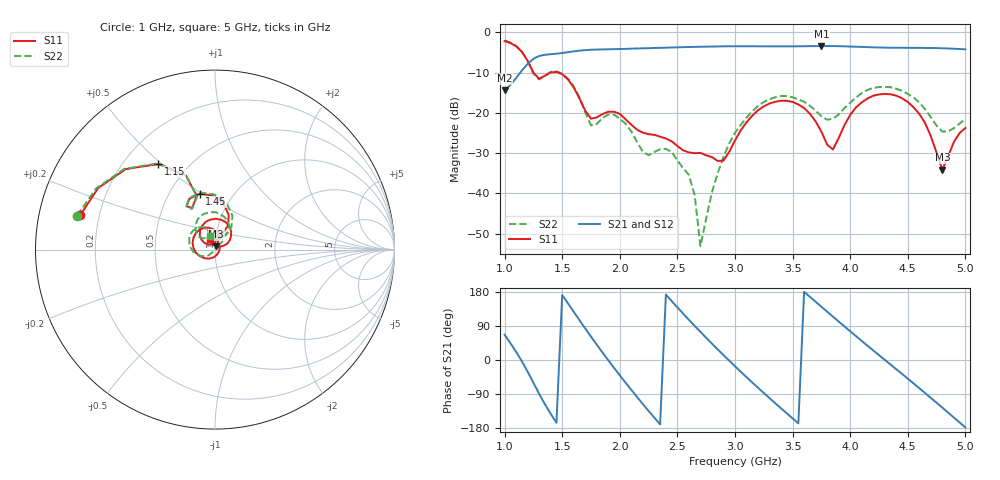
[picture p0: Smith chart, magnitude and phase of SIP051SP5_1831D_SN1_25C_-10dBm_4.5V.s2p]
# GHz  S  dB  R  50
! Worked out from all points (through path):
!   81 points, 1 GHz to 5 GHz, reference 50 ohm
!   highest |S21| = -3.41 dB at 3.75 GHz (marker M1); lowest = -14.4 dB at 1 GHz (marker M2)
!   lowest |S11| = -34.1 dB at 4.8 GHz (marker M3), VSWR 1.04, Z = 50.7 + j1.85 ohm
!   |S11| at or under -10 dB: 1.25 GHz to 1.398 GHz (148 MHz wide, 11.2 % of centre); 1.464 GHz to end of sweep
!   |S22| runs from -53.1 to -2.0 dB; largest |S21 - S12| = 0.0036
!   S11 on the Smith chart (normalised r, x): 1 GHz: 0.13, +0.12; 1.15 GHz: 0.34, +0.49; 1.45 GHz: 0.70, +0.49; 5 GHz: 0.94, +0.11
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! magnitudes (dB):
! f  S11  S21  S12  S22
! 1 GHz  -2.2  -14.4  -14.4  -2.0
! 1.15 GHz  -4.9  -9.5  -9.5  -4.8
! 1.3 GHz  -11.5  -5.9  -5.9  -11.7
! 1.45 GHz  -9.8  -5.3  -5.3  -9.7
! 1.7 GHz  -19.4  -4.4  -4.4  -19.9
! 1.95 GHz  -19.7  -4.2  -4.2  -20.5
! 2.2 GHz  -24.9  -4.0  -4.0  -29.6
! 2.35 GHz  -25.9  -3.9  -3.9  -29.0
! 2.6 GHz  -29.8  -3.7  -3.7  -35.4
! 2.65 GHz  -30.0  -3.6  -3.6  -40.4
! 2.7 GHz  -29.9  -3.6  -3.6  -53.1
! 2.85 GHz  -32.0  -3.5  -3.5  -35.0
! 3 GHz  -26.9  -3.5  -3.5  -25.0
! 3.35 GHz  -17.3  -3.5  -3.5  -16.1
! 3.7 GHz  -22.1  -3.4  -3.4  -19.4
! 3.75 GHz  -24.7  -3.4  -3.4  -20.8
! 3.85 GHz  -29.1  -3.4  -3.4  -21.5
! 4.05 GHz  -18.7  -3.6  -3.6  -16.2
! 4.35 GHz  -15.4  -3.8  -3.8  -13.6
! 4.6 GHz  -20.3  -3.9  -3.9  -17.4
! 4.8 GHz  -34.1  -4.0  -4.0  -24.7
! 5 GHz  -23.8  -4.2  -4.2  -21.6
